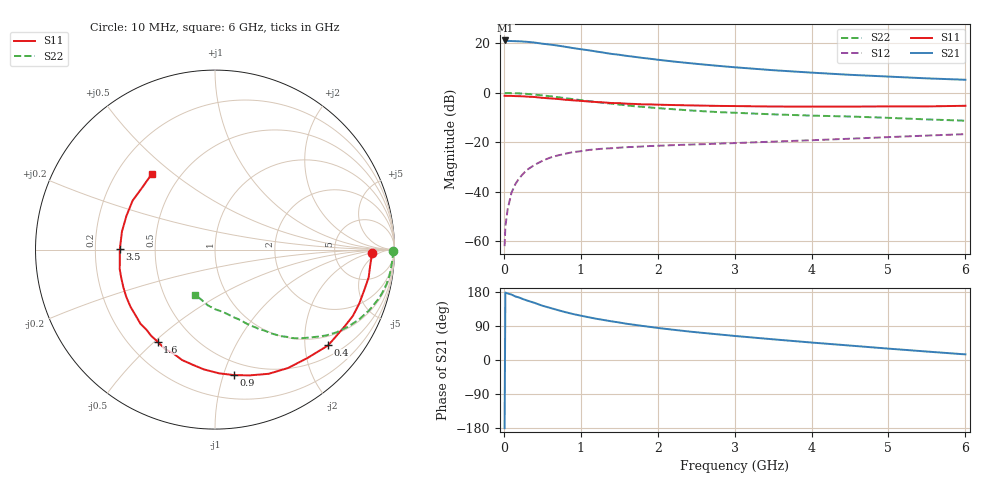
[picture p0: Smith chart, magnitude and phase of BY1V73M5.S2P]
! SIEMENS Small Signal Semiconductors
! BFY420
! Si NPN RF SIEGET Grounded Emitter Transistor in MICRO-X
! VCE = 1.75 V  IC = 3.5 mA
! Common Emitter S-Parameters:  October  1996
# GHz  S  MA  R  50
!  f  S11  S21  S12  S22
! GHz  MAG  ANG  MAG  ANG  MAG  ANG  MAG  ANG
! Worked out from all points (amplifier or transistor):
!   36 points, 10 MHz to 6 GHz, reference 50 ohm
!   highest |S21| = 21.2 dB at 20 MHz (marker M1)
!   |S21| within 3 dB of that: start of sweep to 885.1 MHz
!   unconditionally stable (mu >= 1): 3.453 GHz to end of sweep
!   at 250 MHz: K = 0.08, MSG = 26.7 dB, |S12| = -32.7 dB
!   at 1.4 GHz: K = 0.43, MSG = 19.1 dB, |S12| = -22.4 dB
!   at 6 GHz: K = 1.18, MAG = 8.4 dB, |S12| = -16.7 dB
!   S11 on the Smith chart (normalised r, x): 10 MHz: 14, -3; 400 MHz: 0.76, -2.54; 900 MHz: 0.39, -1.09; 1.6 GHz: 0.32, -0.51; 3.5 GHz: 0.31, +0.00; 6 GHz: 0.35, +0.42
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0.01  0.8744 -1.4  11.43 -179.9  0.0008 101.0  0.9938 -0.5
0.02  0.8742 -2.3  11.47 177.9  0.002 86.6  0.9872 -1.0
0.05  0.8695 -5.3  11.22 175.5  0.0045 86.9  0.9918 -2.7
0.1  0.87 -10.3  11.16 172.7  0.0097 85.5  0.9862 -5.5
0.15  0.8613 -15.5  11.09 167.7  0.0144 80.0  0.9826 -8.4
0.2  0.858 -20.6  11.01 164.8  0.0189 78.2  0.9761 -11.0
0.3  0.8401 -30.4  10.76 157.1  0.0278 73.2  0.9541 -16.4
0.4  0.8261 -40.2  10.38 150.7  0.0351 68.4  0.9238 -21.4
0.5  0.7942 -49.4  9.866 143.3  0.0423 63.3  0.8918 -25.9
0.6  0.7752 -58.3  9.481 137.6  0.0491 59.3  0.8557 -30.2
0.7  0.7539 -66.6  9.044 131.8  0.0544 55.3  0.8194 -34.2
0.9  0.7071 -81.4  8.046 121.3  0.0637 48.6  0.7462 -40.6
1.1  0.6704 -95.3  7.274 112.9  0.0702 43.6  0.6839 -46.3
1.4  0.6237 -111.8  6.134 102.0  0.0762 37.9  0.6064 -52.7
1.6  0.6043 -122.0  5.587 95.5  0.0801 35.0  0.5591 -56.4
2  0.5777 -138.6  4.681 84.6  0.0854 31.1  0.4913 -62.2
2.2  0.5684 -146.0  4.314 79.9  0.0879 29.8  0.4686 -64.8
2.8  0.5455 -163.3  3.502 67.4  0.0946 27.1  0.4081 -71.5
3.5  0.5304 179.8  2.873 54.6  0.1036 25.4  0.3685 -78.5
4.5  0.528 159.1  2.319 38.1  0.1187 22.3  0.3332 -89.4
5.5  0.5333 139.1  1.965 22.3  0.1373 18.4  0.2911 -104.5
6  0.5489 130.1  1.842 14.8  0.1467 15.9  0.2744 -113.6
